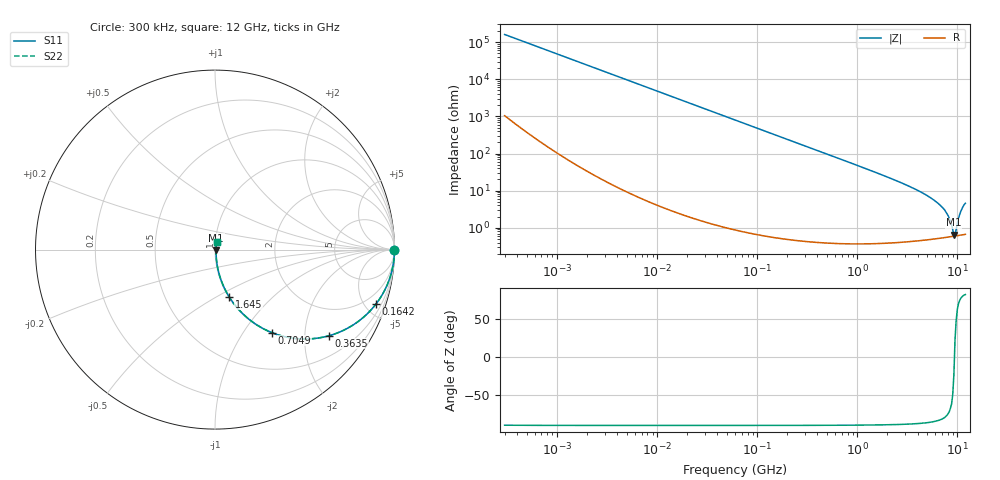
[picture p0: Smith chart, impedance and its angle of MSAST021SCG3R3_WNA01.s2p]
! MSAST021SCG3R3_WNA01  S-PARAMETER MODEL  ( General Type )
! Model Generated by TAIYO YUDEN Corporation (http://www.ty-top.com)
! Version 2.0
! TAIYO YUDEN Control No. 181101
! Copyright(c) 2015 TAIYO YUDEN CO.,LTD. All Rights Reserved.
! Product Description (link to TY-COMPAS)
! https://ds.yuden.co.jp/TYCOMPAS/or/detail?pn=MSAST021SCG3R3BWNA01&u=M
! Products Name : Multilayer Ceramic Capacitors
! Characteristics :
!  Capacitance : 3.3 pF , Rated Voltage : 25V , TCC : CG / C0G
!  Case Size : 0.25 x 0.125 / 0.0098 x 0.0049 [mm/inch] , Thickness : 0.125 / 0.0049 [mm/inch]
!  (Conditions: Temperature = 25 degC , DC Bias Current/Voltage = 0A / 0V)
! External Node Assignments :
!  1  o---| |---o  2
! GND o---------o GND
! Frequency Range : 0.3MHz  -  12000MHz  [ 401 STEP ]
# MHz S RI R 50
! Freq[MHz].  S11 Real  S11 Imag  S21 Real  S21 Imag  S12 Real  S12 Imag  S22 Real  S22 Imag
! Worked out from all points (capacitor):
!   401 points, 300 kHz to 12 GHz, reference 50 ohm
!   read as one part in series: C = 3.3 pF near 316.3 kHz
!   lowest |Z| = 646 mohm at 9.207 GHz (marker M1)
!   series resonance near 9.334 GHz, so ESL is about 88 pH
!   S11 on the Smith chart (normalised r, x): 300 kHz: open; 164.2 MHz: 1.01, -5.87; 363.5 MHz: 1.01, -2.65; 704.9 MHz: 1.01, -1.36; 1.645 GHz: 1.01, -0.57; 12 GHz: 1.01, +0.09
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0.3  1 -0.000622  4.43e-06 0.000622  4.43e-06 0.000622  1 -0.000622
1.769972  1 -0.00367  1.89e-05 0.00367  1.89e-05 0.00367  1 -0.00367
10.44266  0.9995 -0.0216  0.000487 0.0216  0.000487 0.0216  0.9995 -0.0216
60  0.9846 -0.1225  0.0154 0.1225  0.0154 0.1225  0.9846 -0.1225
164.1901  0.8957 -0.3048  0.1043 0.3048  0.1043 0.3048  0.8957 -0.3048
244.3004  0.7951 -0.4025  0.2049 0.4025  0.2049 0.4025  0.7951 -0.4025
353.9943  0.6489 -0.4758  0.3511 0.4758  0.3511 0.4758  0.6489 -0.4758
363.4975  0.6367 -0.4794  0.3633 0.4794  0.3633 0.4794  0.6367 -0.4794
704.9044  0.3177 -0.4629  0.6823 0.4629  0.6823 0.4629  0.3177 -0.4629
1076.992  0.166 -0.3679  0.834 0.3679  0.834 0.3679  0.166 -0.3679
1645.489  0.0782 -0.262  0.9218 0.262  0.9218 0.262  0.0782 -0.262
2088.533  0.0499 -0.2092  0.9501 0.2092  0.9501 0.2092  0.0499 -0.2092
4050.141  0.0142 -0.0982  0.9858 0.0982  0.9858 0.0982  0.0142 -0.0982
6188.031  0.00739 -0.0482  0.9926 0.0482  0.9926 0.0482  0.00739 -0.0482
7648.807  0.00613 -0.0258  0.9939 0.0258  0.9939 0.0258  0.00613 -0.0258
8281.503  0.00593 -0.0171  0.9941 0.0171  0.9941 0.0171  0.00593 -0.0171
8966.534  0.00587 -0.00681  0.9941 0.00681  0.9941 0.00681  0.00587 -0.00681
9207.246  0.00589 -0.00256  0.9941 0.00256  0.9941 0.00256  0.00589 -0.00256
9708.23  0.00607 0.00653  0.9939 -0.00653  0.9939 -0.00653  0.00607 0.00653
10511.28  0.0067 0.0214  0.9933 -0.0214  0.9933 -0.0214  0.0067 0.0214
11083.22  0.00737 0.0313  0.9926 -0.0313  0.9926 -0.0313  0.00737 0.0313
12000  0.00862 0.0445  0.9914 -0.0445  0.9914 -0.0445  0.00862 0.0445
